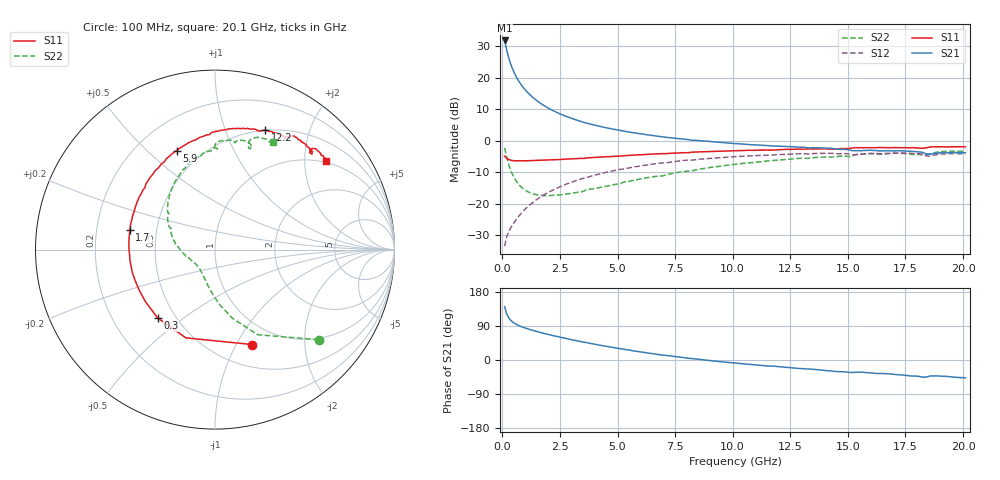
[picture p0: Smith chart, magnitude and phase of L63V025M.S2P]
!  Infineon Technologies AG
! BFR380L3 , PF131585-7, No.6, Th 09.10.01, soldered on pcb-board, measured with PP GSG850
!  Vce=3.0 V,  Ic=25.0 mA
! Common Emitter S-Parameters:  15. November 2001
#  GHz  S  MA  R  50
! f  S11  S21  S12  S22
! GHz  Mag  Ang  Mag  Ang  Mag  Ang  Mag  Ang
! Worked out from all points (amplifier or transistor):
!   201 points, 100 MHz to 20.1 GHz, reference 50 ohm
!   highest |S21| = 31.8 dB at 100 MHz (marker M1)
!   |S21| within 3 dB of that: start of sweep to 190.5 MHz
!   unconditionally stable (mu >= 1): 1.332 GHz to 4.311 GHz
!   at 3.4 GHz: K = 1.02, MAG = 8.4 dB, |S12| = -12.2 dB
!   at 10.1 GHz: K = 0.96, MSG = 2.1 dB, |S12| = -5.1 dB
!   at 20.1 GHz: K = 0.99, MSG = 0.1 dB, |S12| = -4.1 dB
!   S11 on the Smith chart (normalised r, x): 100 MHz: 0.75, -1.16; 300 MHz: 0.40, -0.40; 1.7 GHz: 0.35, +0.10; 5.9 GHz: 0.37, +0.62; 12.2 GHz: 0.50, +1.38; 20.1 GHz: 0.95, +2.53
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0.1  0.5677 -68.7  38.76 140.7  0.02107 62.7  0.7653 -41.0
0.2  0.5179 -108.3  26.46 120.1  0.03055 56.1  0.5305 -63.3
0.3  0.4972 -129.9  19.32 109.5  0.03708 55.9  0.394 -75.9
0.4  0.4841 -143.3  15.05 102.7  0.04323 56.9  0.3135 -84.4
0.5  0.4789 -152.4  12.27 98.0  0.04925 59.1  0.2626 -91.0
0.6  0.4772 -159.2  10.33 94.4  0.05565 60.5  0.2284 -96.4
0.7  0.4781 -164.4  8.932 91.3  0.06194 61.9  0.2035 -101.3
0.8  0.4762 -168.9  7.859 88.7  0.06863 63.1  0.1858 -105.5
1  0.4768 -176.1  6.345 84.2  0.08204 64.3  0.1624 -112.9
1.2  0.4793 178.2  5.32 80.3  0.09544 65.0  0.1487 -119.4
1.4  0.4824 173.6  4.588 76.8  0.1093 65.1  0.1405 -125.1
1.7  0.4867 167.2  3.809 71.9  0.13 64.6  0.1348 -132.7
2.4  0.4987 154.7  2.759 61.6  0.178 61.9  0.1356 -146.9
3.5  0.5204 138.7  1.961 47.4  0.2511 55.5  0.1553 -163.0
4.5  0.5527 126.2  1.597 36.1  0.3129 49.0  0.1883 -177.8
5.9  0.5918 111.2  1.295 22.2  0.3909 39.5  0.2417 165.3
6.8  0.6165 102.5  1.165 14.2  0.4357 32.9  0.2732 154.8
10.1  0.6885 78.3  0.8949 -7.9  0.5544 11.4  0.4189 124.7
12.2  0.7208 67.3  0.8071 -18.9  0.6035 -1.3  0.4983 107.4
13.5  0.733 60.7  0.77 -24.7  0.6196 -9.2  0.5328 98.2
16.8  0.7715 48.4  0.6895 -36.4  0.6266 -25.0  0.6218 77.6
20.1  0.7917 38.7  0.6413 -47.1  0.6204 -38.6  0.6795 61.7
